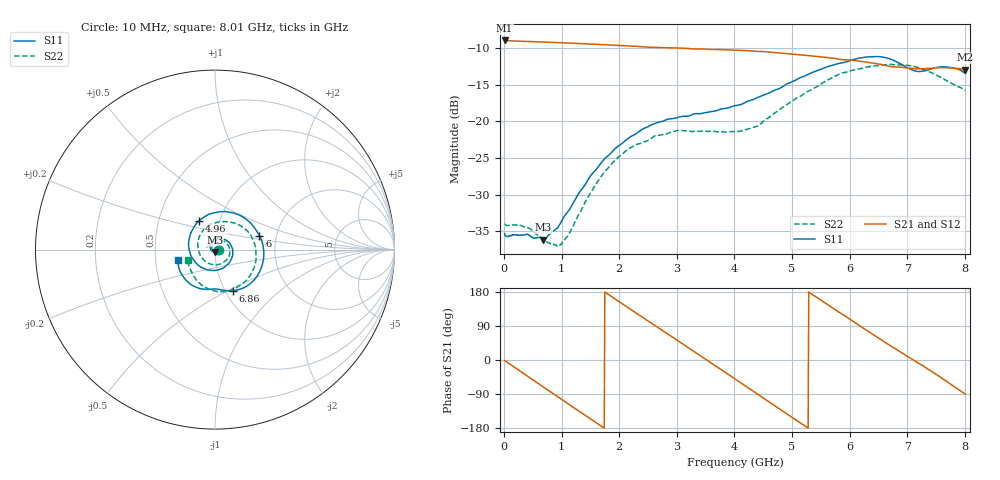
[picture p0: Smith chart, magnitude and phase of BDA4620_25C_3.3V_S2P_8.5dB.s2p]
!Agilent Technologies,E5071B,MY42404982,A.09.10
!Date: Wed May 06 08:50:11 2026
!Data & Calibration Information:
!Freq	S11:SOLT2(ON)	S21:SOLT2(ON)	S12:SOLT2(ON)	S22:SOLT2(ON)
# Hz S RI R 50
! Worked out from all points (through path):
!   801 points, 10 MHz to 8.01 GHz, reference 50 ohm
!   highest |S21| = -8.94 dB at 10 MHz (marker M1); lowest = -12.9 dB at 8.01 GHz (marker M2)
!   group delay of S21, straight-line fit = 281 ps
!   lowest |S11| = -36.2 dB at 680 MHz (marker M3), VSWR 1.03, Z = 49.8 - j1.54 ohm
!   |S11| at or under -10 dB: start of sweep to end of sweep
!   |S22| runs from -37.1 to -12.2 dB; largest |S21 - S12| = 0.0016
!   S11 on the Smith chart (normalised r, x): 10 MHz: 1.03, -0.00; 4.96 GHz: 0.80, +0.26; 6 GHz: 1.63, +0.27; 6.86 GHz: 1.08, -0.53; 8.01 GHz: 0.66, -0.08
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1e7  0.017 -0.00125  0.3571 -0.00774  0.3574 -0.00764  0.0199 -0.00123
3.2e8  0.0131 -0.0104  0.2934 -0.1951  0.2938 -0.1956  0.0168 -0.00949
6.8e8  -0.00157 -0.0155  0.1138 -0.3293  0.1138 -0.33  0.00367 -0.0152
9.8e8  -0.0189 -0.00677  -0.071 -0.3375  -0.0715 -0.3378  -0.0115 -0.00856
1.35e9  -0.0263 0.0222  -0.2601 -0.2186  -0.2603 -0.2189  -0.0198 0.0155
1.65e9  -0.0105 0.0487  -0.3305 -0.0549  -0.3311 -0.0548  -0.00959 0.0388
1.94e9  0.021 0.0623  -0.3108 0.1138  -0.3111 0.1143  0.0154 0.0526
2.32e9  0.0695 0.0468  -0.1679 0.2782  -0.1684 0.2787  0.0551 0.043
2.68e9  0.0985 -0.00161  0.0279 0.3189  0.0282 0.3192  0.0796 0.01
3e9  0.0886 -0.0579  0.1923 0.2523  0.1928 0.2524  0.0804 -0.0315
3.39e9  0.0338 -0.1075  0.3043 0.0716  0.3048 0.0714  0.0429 -0.0737
3.69e9  -0.0287 -0.1149  0.2961 -0.0915  0.2961 -0.0922  -0.00441 -0.0848
4.01e9  -0.0961 -0.0844  0.1972 -0.2347  0.1974 -0.2352  -0.0577 -0.0629
4.48e9  -0.1473 0.0279  -0.0417 -0.2972  -0.0419 -0.2977  -0.0957 0.0219
4.96e9  -0.0892 0.1604  -0.2432 -0.1568  -0.2441 -0.1567  -0.0438 0.1268
5.35e9  0.0393 0.2121  -0.2775 0.0328  -0.2778 0.0328  0.0581 0.1551
6e9  0.2475 0.0785  -0.0814 0.2504  -0.0817 0.2506  0.2163 0.0444
6.34e9  0.2661 -0.0743  0.071 0.2421  0.0716 0.2424  0.2271 -0.0663
6.68e9  0.1727 -0.2063  0.1822 0.1535  0.1828 0.1537  0.1743 -0.1716
6.86e9  0.099 -0.2296  0.2155 0.0937  0.2161 0.0935  0.1252 -0.2086
7.42e9  -0.0567 -0.2213  0.2008 -0.1134  0.2011 -0.1142  -0.0619 -0.2055
8.01e9  -0.2053 -0.057  -0.000761 -0.226  -0.000637 -0.2266  -0.1517 -0.0602
